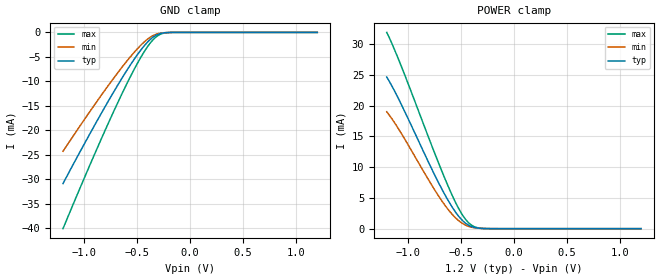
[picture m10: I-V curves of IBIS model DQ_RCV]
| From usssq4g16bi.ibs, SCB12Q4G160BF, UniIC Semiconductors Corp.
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|   Model DQ_RCV
[Model] DQ_RCV
Model_type Input
Polarity   Non-Inverting
Enable   Active-High
Vinl =  8.300E-01
Vinh =  9.700E-01
C_comp   8.561E-13   8.432E-13   8.711E-13
C_comp_power_clamp   3.173E-13   3.072E-13   3.290E-13
C_comp_gnd_clamp   5.388E-13   5.359E-13   5.421E-13
[Model Spec]
Vinh   9.700E-01   9.250E-01   1.015E+00
Vinl   8.300E-01   7.850E-01   8.750E-01
[Temperature Range]   45.000   95.000   -40.000
[Voltage Range]   1.200E+00   1.140E+00   1.260E+00
[C Comp Corner]
C_comp_power_clamp   3.173E-13   3.290E-13   3.072E-13
C_comp_gnd_clamp   5.388E-13   5.421E-13   5.359E-13
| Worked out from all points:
|   GND clamp passes 1 mA (typ) near -0.35 V on its own axis
|   POWER clamp passes 1 mA (typ) near -0.46 V on its own axis
[GND_clamp]
|Voltage   I(typ)   I(min)   I(max)
-1.2V     -30.84mA   -24.25mA   -40.04mA
-875mV    -17.92mA   -13.94mA   -23.52mA
-750mV    -13.19mA   -10.17mA   -17.47mA
-625mV    -8.699mA   -6.602mA   -11.7mA
-525mV    -5.384mA   -3.989mA   -7.412mA
-450mV    -3.179mA   -2.281mA   -4.518mA
-375mV    -1.408mA   -958.6uA   -2.123mA
-325mV    -614.2uA   -404.9uA   -980.6uA
-250mV    -97.6uA    -67.88uA   -160.7uA
-175mV    -8.82uA    -7.635uA   -12.18uA
1.2V      0A         0A         0A
[POWER_clamp]
|Voltage   I(typ)   I(min)   I(max)
-1.2V     24.65mA    19.01mA    31.9mA
-1.15V    23.15mA    17.82mA    30.04mA
-1.075V   20.62mA    15.83mA    26.93mA
-775mV    9.691mA    7.064mA    13.48mA
-625mV    4.722mA    3.212mA    7.078mA
-550mV    2.672mA    1.744mA    4.238mA
-500mV    1.586mA    1.017mA    2.629mA
-450mV    802uA      518.6uA    1.374mA
-400mV    337uA      230.9uA    568.8uA
-350mV    119.1uA    91.13uA    183.1uA
-250mV    9.454uA    10.16uA    10.01uA
1.2V      0A         0A         2.743nA
